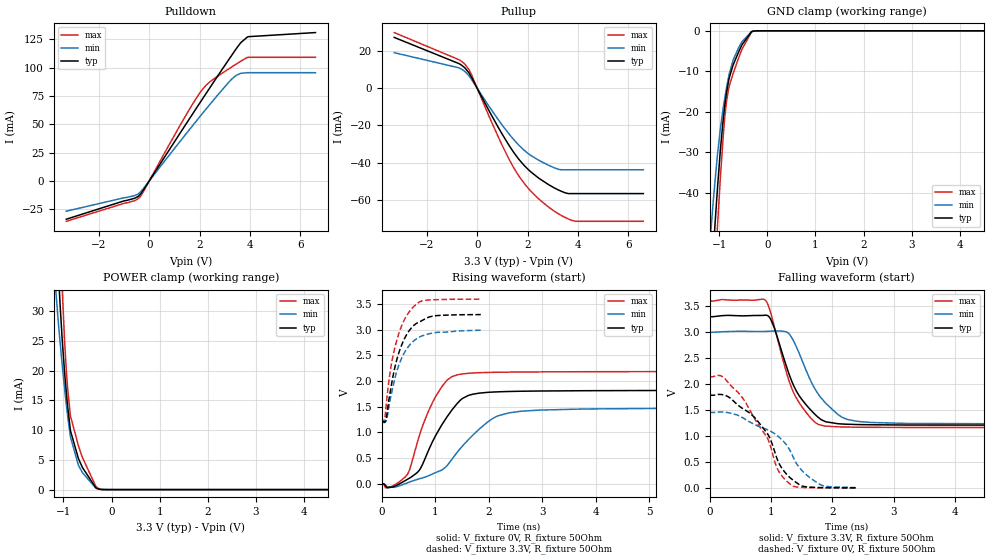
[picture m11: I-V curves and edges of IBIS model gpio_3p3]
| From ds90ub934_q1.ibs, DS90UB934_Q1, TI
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|   gpio_3p3 Model
[Model]   gpio_3p3
Model_type   I/O
Polarity   Non-Inverting
Enable   Active-Low
Vinl = 0.8
Vinh = 2
Vmeas = 1.65
Vref = 0
Cref = 2pF
Rref = 100
|   typ   min   max
|   (nom PVT)   (fast PVT)   (slow PVT)
C_comp   3.371e-13   3.361e-13   3.845e-13
| Where nom  PVT is Nominal Process, 3.3V, 27C
|   Fast PVT is Strong Process,  3.6V, -40C
|   Slow PVT is Weak Process,   3V, 125C
[Voltage Range]   3.3   3   3.6
|Junction Temperature
[Temperature Range]   27   125   -40
[Pullup Reference]   3.3   3   3.6
[Pulldown Reference]   0   0   0
[Power Clamp Reference]   3.3   3   3.6
[GND Clamp Reference]   0   0   0
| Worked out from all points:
|   slope of the pulldown table from 0 to 0.495 V, typ, clamps not added: 29 ohm
|   slope of the pullup table from 0 to 0.495 V, typ, clamps not added: 38.9 ohm
|   GND clamp passes 1 mA (typ) near -0.38 V on its own axis
|   falling waveform, V_fixture 3.3V, R_fixture 50Ohm: 20-80 % time 444ps typ, 490ps min, 388ps max; typ from 3.3 V to 1.21 V
|   rising waveform, V_fixture 0V, R_fixture 50Ohm: 20-80 % time 558ps typ, 789ps min, 456ps max; typ from 0 V to 1.8 V
|   rising waveform, V_fixture 3.3V, R_fixture 50Ohm: 20-80 % time 319ps typ, 328ps min, 291ps max; typ from 1.21 V to 3.3 V
|   falling waveform, V_fixture 0V, R_fixture 50Ohm: 20-80 % time 526ps typ, 688ps min, 536ps max; typ from 1.79 V to 0.001 V
[Pulldown]
|   Voltage   I(typ)   I(min)   I(max)
-3.3V     -33.8mA    -26.73mA   -35.63mA
-621mV    -15.55mA   -13.2mA    -17.7mA
-416.4mV  -13.15mA   -11.02mA   -15.19mA
-243.6mV  -8.298mA   -6.901mA   -9.764mA
1.479V    50.9mA     42.06mA    58.86mA
2.057V    70.47mA    58.02mA    79.16mA
2.436V    83.19mA    68.27mA    87.87mA
3.303V    111.7mA    90.39mA    100.9mA
3.623V    121.6mA    94.78mA    105.4mA
3.871V    126.5mA    95.44mA    108.7mA
3.925V    127.2mA    95.44mA    109mA
6.6V      130.8mA    95.44mA    109mA
[GND Clamp]
|   Voltage   I(typ)   I(min)   I(max)
-3.3V     -491.8mA   -423.9mA   -559.8mA
-1.239V   -75.42mA   -59.14mA   -91.74mA
-1.131V   -55.26mA   -42.87mA   -68mA
-1.118V   -52.97mA   -41.09mA   -65.28mA
-1.035V   -38.5mA    -30.32mA   -47.74mA
-916.8mV  -21.68mA   -18.91mA   -25.82mA
-858mV    -16mA      -14.63mA   -18.24mA
-808.8mV  -12.51mA   -11.55mA   -14.49mA
-711mV    -8.408mA   -7.158mA   -10.49mA
-597mV    -5.192mA   -4.144mA   -6.684mA
-330mV    -214.7uA   -206.3uA   -301.9uA
6.6V      0A         0A         0A
[Pullup]
|   Voltage   I(typ)   I(min)   I(max)
-3.3V     27.38mA    19.16mA    29.98mA
-726mV    13.26mA    10.98mA    15.37mA
-495mV    11.02mA    9.082mA    13.04mA
-214.8mV  5.559mA    4.494mA    6.876mA
858mV     -21.64mA   -17.37mA   -26.91mA
1.461V    -34.78mA   -27.84mA   -43.1mA
2.13V     -45.07mA   -36.2mA    -55.48mA
2.883V    -52.3mA    -41.79mA   -64.48mA
3.245V    -54.91mA   -43.73mA   -67.77mA
3.513V    -56.41mA   -43.89mA   -69.71mA
3.92V     -56.73mA   -43.89mA   -71.65mA
6.6V      -56.73mA   -43.89mA   -71.65mA
[POWER Clamp]
|   Voltage   I(typ)   I(min)   I(max)
-3.3V     582.6mA    466.3mA    697.7mA
-1.155V   45.95mA    33.1mA     64.9mA
-1.089V   34.1mA     26.51mA    48.26mA
-1.072V   31.39mA    24.93mA    44.12mA
-1.023V   24.87mA    20.75mA    33.46mA
-1.014V   23.81mA    20.01mA    31.67mA
-975mV    19.64mA    16.9mA     24.86mA
-937.2mV  16.08mA    14.08mA    19.71mA
-852mV    9.838mA    8.778mA    12.31mA
-660mV    4.699mA    3.657mA    6.688mA
-306.9mV  228.3uA    200.3uA    413.1uA
6.6V      0A         0A         0A
[Ramp]
R_load = 50
|   typ   min   max
dV/dt_r   1.07754/5.57178e-10   0.880333/7.80725e-10  1.29209/4.54918e-10
dV/dt_f   1.25195/4.43147e-10   1.0571/4.86178e-10   1.43998/3.87318e-10
[Falling Waveform]
V_fixture = 3.3V
V_fixture_min = 3V
V_fixture_max = 3.6V
R_fixture = 50Ohm
|   Time   V(typ)   V(min)   V(max)
0s        3.3V       3V         3.6V
911.5ps   3.328V     3.016V     3.612V
1.037ns   3.133V     3.023V     3.186V
1.252ns   2.34V      3.005V     2.222V
1.413ns   1.867V     2.719V     1.732V
1.75ns    1.38V      1.843V     1.239V
2.086ns   1.237V     1.419V     1.177V
2.38ns    1.222V     1.287V     1.17V
3.221ns   1.212V     1.242V     1.165V
39.35ns   1.213V     1.237V     1.199V
[Rising Waveform]
V_fixture = 0V
V_fixture_min = 0V
V_fixture_max = 0V
R_fixture = 50Ohm
|   Time   V(typ)   V(min)   V(max)
0s        975nV      4.518uV    2.409uV
133.5ps   -66.43mV   -75.67mV   -75.59mV
483.2ps   88.32mV    19.26mV    187.9mV
841.1ps   567.4mV    141.6mV    1.334V
1.221ns   1.304V     351.6mV    2.018V
1.515ns   1.666V     742mV      2.141V
2.032ns   1.785V     1.241V     2.171V
2.95ns    1.808V     1.436V     2.18V
7.921ns   1.821V     1.476V     2.187V
100ns     1.796V     1.467V     2.153V
[Rising Waveform]
V_fixture = 3.3V
V_fixture_min = 3V
V_fixture_max = 3.6V
R_fixture = 50Ohm
|   Time   V(typ)   V(min)   V(max)
0s        1.213V     1.238V     1.2V
46.2ps    1.203V     1.237V     1.195V
80.35ps   1.244V     1.228V     1.501V
154.8ps   1.763V     1.627V     2.163V
265.9ps   2.356V     2.136V     2.739V
379.1ps   2.721V     2.464V     3.096V
548.9ps   3.031V     2.735V     3.399V
719.8ps   3.162V     2.866V     3.551V
990ps     3.273V     2.945V     3.586V
1.853ns   3.297V     2.993V     3.598V
[Falling Waveform]
V_fixture = 0V
V_fixture_min = 0V
V_fixture_max = 0V
R_fixture = 50Ohm
|   Time   V(typ)   V(min)   V(max)
0s        1.786V     1.454V     2.144V
243.2ps   1.787V     1.459V     2.111V
535.8ps   1.531V     1.355V     1.735V
721.6ps   1.37V      1.228V     1.358V
955.4ps   1.019V     1.115V     923.1mV
1.116ns   510.5mV    993.2mV    341mV
1.315ns   191.7mV    708.1mV    69.07mV
1.504ns   37.06mV    333.8mV    8.848mV
1.796ns   6.572mV    66.51mV    2.073mV
2.38ns    1.093mV    5.381mV    722.9uV
